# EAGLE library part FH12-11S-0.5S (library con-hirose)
0.5mm Pitch Connectors For FPC/FFC Source: Data sheet
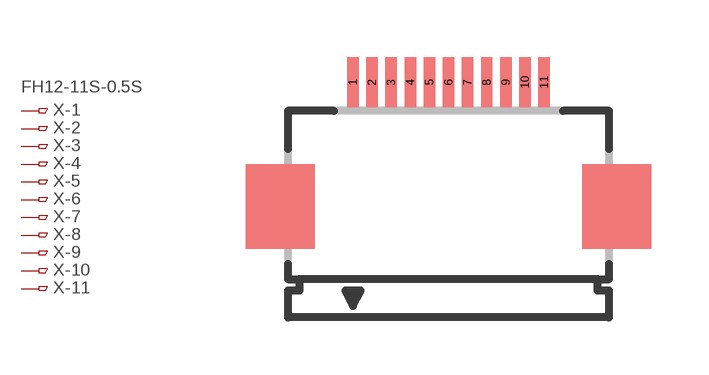
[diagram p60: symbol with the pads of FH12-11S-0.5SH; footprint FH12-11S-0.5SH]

Designator prefix X; gates -1=PINV -2=PIN -3=PIN -4=PIN -5=PIN -6=PIN -7=PIN -8=PIN -9=PIN -10=PIN -11=PIN

## FH12-11S-0.5SH (OC_FARNELL: 1324541; OC_NEWARK: unknown)  [FH12-11S-0.5SH]
1  -1:1  pas
2  -2:1  pas
3  -3:1  pas
4  -4:1  pas
5  -5:1  pas
6  -6:1  pas
7  -7:1  pas
8  -8:1  pas
9  -9:1  pas
10  -10:1  pas
11  -11:1  pas

## Footprint FH12-11S-0.5SH (pad centres in mm)
0.5mm Pitch Connectors For FPC/FFC Source: Data sheet
smd 0.3 x 1.3: 1 -2.5,3.25; 2 -2,3.25; 3 -1.5,3.25; 4 -1,3.25; 5 -0.5,3.25; 6 0,3.25; 7 0.5,3.25; 8 1,3.25; 9 1.5,3.25; 10 2,3.25; 11 2.5,3.25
